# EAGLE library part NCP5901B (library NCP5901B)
The NCP5901B is a high performance dual MOSFET gate driver optimized to drive the gates of both high−side and low−side power MOSFETs in a synchronous buck converter.
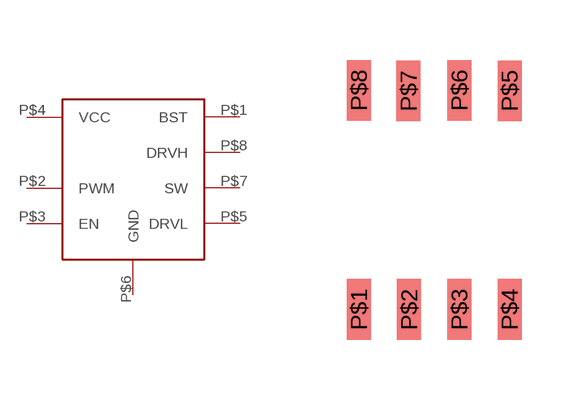
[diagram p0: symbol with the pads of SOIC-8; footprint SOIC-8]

Designator prefix -

## NCP5901B  [SOIC-8]
P$1  BST
P$2  PWM  in
P$3  EN  in
P$4  VCC  pwr
P$5  DRVL  out
P$6  GND  pwr
P$7  SW
P$8  DRVH  out

## Footprint SOIC-8 (pad centres in mm)
smd 0.6 x 1.52: P$1 0.305,1.092; P$2 1.562,1.092; P$3 2.819,1.092; P$4 4.077,1.092; P$5 4.077,6.566; P$6 2.819,6.579; P$7 1.549,6.566; P$8 0.305,6.579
